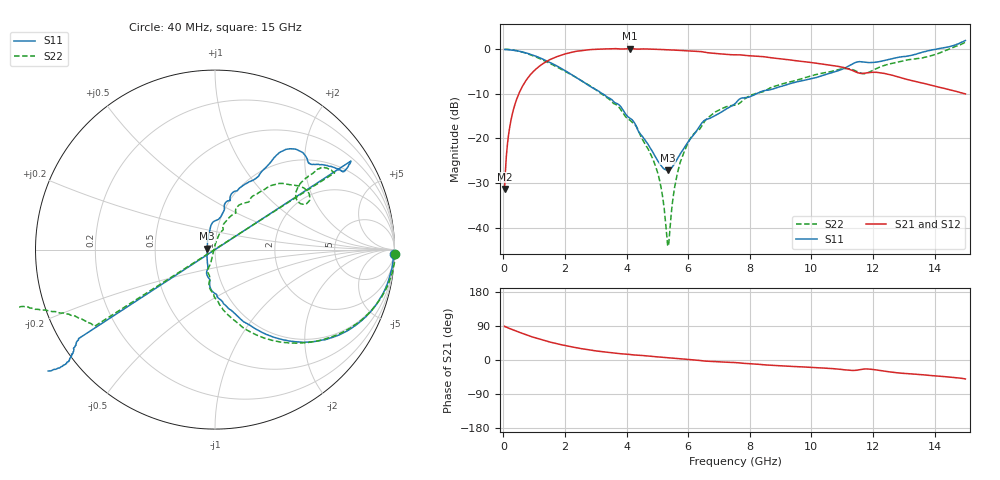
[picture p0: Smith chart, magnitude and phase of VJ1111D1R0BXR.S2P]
! VJ1111D1R0BXR
! DATE 03/08/2022  10:31
! CAPACITORS MOUNTED IN SERIES ON 25 MIL THICK MICROSTRIP SUBSTRATE
# GHz  S  MA  R  50.00
!  FREQ  S11M  S11A  S21M  S21A  S12M  S12A  S22M  S22A
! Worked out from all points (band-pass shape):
!   801 points, 40 MHz to 15 GHz, reference 50 ohm
!   highest |S21| = 0.18 dB at 4.117 GHz (marker M1); lowest = -31.3 dB at 40 MHz (marker M2)
!   |S21| within 3 dB of the highest: 1.372 GHz to 9.838 GHz (8.466 GHz wide, 151 % of centre)
!   lowest |S11| = -27.2 dB at 5.332 GHz (marker M3), VSWR 1.09, Z = 45.8 + j0.489 ohm
!   |S11| at or under -10 dB: 3.231 GHz to 8.207 GHz (4.976 GHz wide, 87 % of centre)
!   |S22| runs from -44.2 to 1.6 dB; largest |S21 - S12| = 0.0057
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0.04  0.9965 -1.5  0.02708 89.1  0.02589 87.7  1.005 -1.5
0.1522  0.9919 -5.4  0.09946 84.9  0.09934 84.9  0.9987 -5.5
0.2644  0.9839 -9.4  0.1715 81.1  0.1715 81.0  0.9899 -9.4
0.6758  0.924 -23.3  0.4155 68.3  0.4152 68.3  0.9197 -23.5
1.4425  0.7337 -44.6  0.7449 48.9  0.7434 48.9  0.715 -46.6
2.5458  0.4444 -67.2  0.9666 29.7  0.9647 29.8  0.4412 -71.7
4.1166  0.1682 -100.2  1.021 14.5  1.018 14.6  0.1596 -100.2
4.7337  0.08179 -121.4  1.009 10.1  1.006 10.3  0.07196 -108.0
5.0329  0.05475 -144.5  0.999 8.1  0.9965 8.2  0.03882 -112.4
5.3321  0.04384 173.0  0.9884 6.1  0.987 6.2  0.006336 -176.3
5.3882  0.04458 164.5  0.9868 5.8  0.9856 5.9  0.007939 125.3
5.65  0.05927 135.1  0.9796 4.0  0.9778 4.1  0.04073 83.6
6.024  0.09427 110.9  0.9625 1.3  0.9614 1.4  0.09362 73.3
6.8094  0.1757 82.0  0.9061 -3.9  0.903 -3.8  0.1897 66.8
7.52  0.246 77.9  0.8689 -6.7  0.8674 -6.6  0.2363 60.5
10.0258  0.4715 59.5  0.7091 -19.5  0.7062 -19.3  0.5075 46.4
11.5405  0.7275 48.4  0.5428 -26.1  0.5408 -26.0  0.5523 27.2
12.5129  0.7707 37.7  0.5244 -31.1  0.5232 -30.9  0.6817 38.0
13.4105  0.8887 32.4  0.4334 -37.6  0.4326 -37.4  0.7859 33.9
13.5788  0.9247 -146.3  0.42 -38.8  0.4184 -38.4  0.8017 -148.6
14.5138  1.078 -142.7  0.3499 -45.0  0.3497 -44.8  1.023 -160.7
15  1.26 -147.2  0.3163 -50.0  0.317 -49.5  1.206 -165.0
